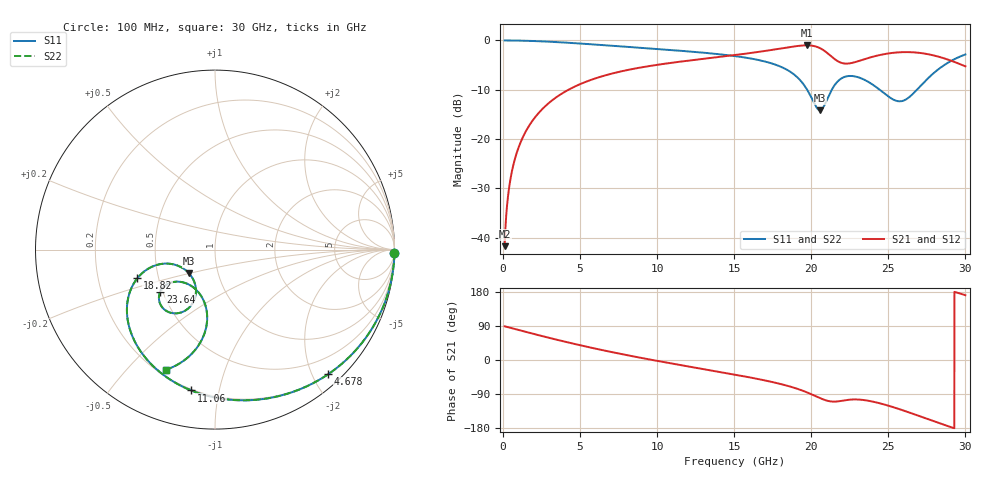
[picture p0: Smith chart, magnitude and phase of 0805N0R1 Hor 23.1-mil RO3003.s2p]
# GHz S MA R 50
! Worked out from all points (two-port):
!   3201 points, 100 MHz to 30 GHz, reference 50 ohm
!   highest |S21| = -0.99 dB at 19.7 GHz (marker M1); lowest = -41.7 dB at 100 MHz (marker M2)
!   |S21| within 3 dB of the highest: 12.29 GHz to 21.61 GHz (9.315 GHz wide, 54.9 % of centre); 23.26 GHz to 28.97 GHz (5.714 GHz wide, 21.9 % of centre)
!   lowest |S11| = -14.2 dB at 20.56 GHz (marker M3), VSWR 1.49, Z = 36.2 - j9.95 ohm
!   |S11| at or under -10 dB: 19.73 GHz to 21.33 GHz (1.595 GHz wide, 7.77 % of centre); 24.44 GHz to 26.85 GHz (2.408 GHz wide, 9.39 % of centre)
!   |S22| runs from -14.2 to 0.0 dB; largest |S21 - S12| = 0
!   S11 on the Smith chart (normalised r, x): 100 MHz: open; 4.678 GHz: 0.19, -2.24; 11.06 GHz: 0.19, -0.83; 18.82 GHz: 0.38, -0.15; 23.64 GHz: 0.48, -0.27; 30 GHz: 0.23, -0.65
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0.1  1 -1.1  0.008227 88.9  0.008227 88.9  1 -1.1
0.3335938  0.9996 -3.6  0.02743 86.4  0.02743 86.4  0.9996 -3.6
0.5391563  0.999 -5.8  0.04428 84.2  0.04428 84.2  0.999 -5.8
1.305344  0.9942 -13.9  0.1063 76.0  0.1063 76.0  0.9942 -13.9
2.650844  0.9772 -27.9  0.2094 61.9  0.2094 61.9  0.9772 -27.9
4.678438  0.9378 -47.8  0.3426 42.0  0.3426 42.0  0.9378 -47.8
5.089563  0.9287 -51.6  0.3659 38.1  0.3659 38.1  0.9287 -51.6
7.406813  0.876 -71.7  0.4759 17.9  0.4759 17.9  0.876 -71.7
10.06978  0.8174 -92.3  0.5683 -2.8  0.5683 -2.8  0.8174 -92.3
11.06022  0.7959 -99.5  0.5973 -10.1  0.5973 -10.1  0.7959 -99.5
15.05  0.6941 -128.0  0.7116 -38.6  0.7116 -38.6  0.6941 -128.0
18.81553  0.4604 -159.8  0.8665 -72.4  0.8665 -72.4  0.4604 -159.8
19.70319  0.3217 -165.2  0.8923 -85.1  0.8923 -85.1  0.3217 -165.2
20.03956  0.2576 -162.0  0.8854 -91.0  0.8854 -91.0  0.2576 -162.0
20.56281  0.196 -137.6  0.836 -100.5  0.836 -100.5  0.196 -137.6
21.17016  0.2829 -112.8  0.717 -108.7  0.717 -108.7  0.2829 -112.8
21.97372  0.4142 -121.0  0.5916 -107.7  0.5916 -107.7  0.4142 -121.0
23.63691  0.3855 -142.4  0.6595 -107.1  0.6595 -107.1  0.3855 -142.4
25.01978  0.2694 -138.4  0.7392 -120.7  0.7392 -120.7  0.2694 -138.4
26.04759  0.248 -114.7  0.762 -134.2  0.762 -134.2  0.248 -114.7
27.51456  0.405 -96.3  0.7286 -155.4  0.7286 -155.4  0.405 -96.3
30  0.7215 -112.1  0.5464 171.1  0.5464 171.1  0.7215 -112.1
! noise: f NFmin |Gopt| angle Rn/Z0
0.1  0.004697  0.9919  0.9887  0.1335
3.417  0.01536  0.875  22.37  0.02554
6.743  0.0217  0.8293  41.62  0.02343
10.06  0.02634  0.7993  59.77  0.02052
13.39  0.02884  0.7688  76.87  0.01576
16.7  0.02905  0.7291  92.71  0.01045
20.03  0.09362  0.8915  105.1  0.06981
23.35  0.2355  0.9495  118.8  0.2716
26.67  0.1872  0.9294  131.8  0.09894
30  0.1997  0.9266  144  0.05835
